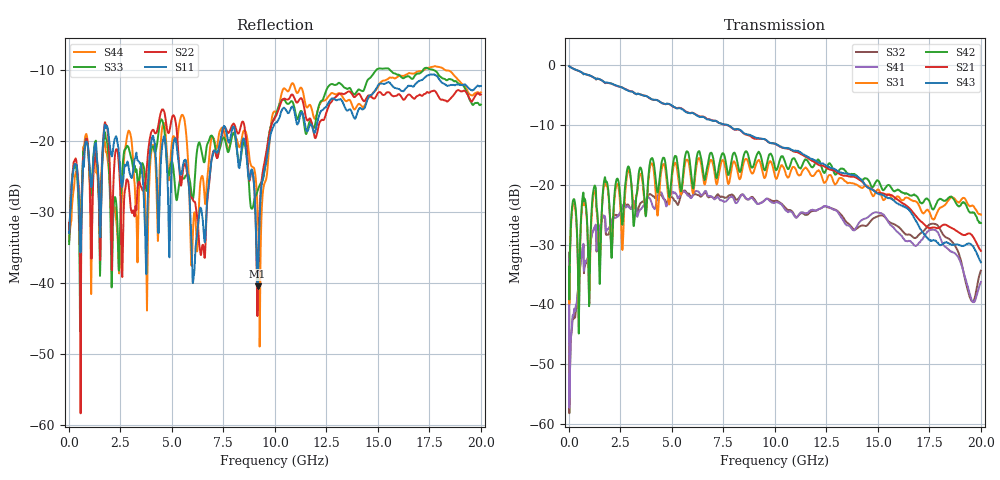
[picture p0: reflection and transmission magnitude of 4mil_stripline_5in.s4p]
! FILE: C:\Archive\Backplane\4-mil striplines\4mil_stripline_5in.s4p
! SMA ->1inch 21mil width microstrip -> 5 inch 4-mil width stripline -> 1 inch 21mil width microstrip -> SMA
! Port 1 -> Port 2, Port 3 -> Port 4
! 10/8/08
# MHz S DB R 50.00
! FREQ  S11  S12  S13  S14
!  S21  S22  S23  S24
!  S31  S32  S33  S34
!  S41  S42  S43  S44
!  DB  ANG  DB  ANG  DB  ANG  DB  ANG
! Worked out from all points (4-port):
!   2000 points, 10 MHz to 20 GHz, reference 50 ohm
!   strongest paths, dB at 10 MHz, 5.01 GHz, 10.01 GHz, 15.01 GHz, 20 GHz:
!     S43: -0.2, -6.8, -13.1, -21.5, -33.0
!     S21: -0.2, -6.8, -13.2, -21.4, -31.0
!     S42: -33.7, -17.7, -17.3, -19.3, -26.4
!     S31: -34.4, -18.5, -18.7, -20.8, -25.0
!     S41: -32.4, -21.3, -23.0, -24.6, -36.2
!     S32: -31.4, -22.1, -22.7, -25.2, -34.4
!   lowest |S11| = -40.5 dB at 9.16 GHz (marker M1), VSWR 1.02, Z = 49.1 - j0.0878 ohm
!   |S11| at or under -10 dB: start of sweep to end of sweep
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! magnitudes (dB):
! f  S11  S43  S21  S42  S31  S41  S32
! 10 MHz  -32.8  -0.2  -0.2  -33.7  -34.4  -32.4  -31.4
! 4.55 GHz  -20.1  -6.4  -6.4  -15.6  -16.7  -21.8  -22.1
! 6.51 GHz  -31.5  -8.7  -8.6  -17.8  -18.7  -21.6  -21.7
! 8.43 GHz  -19.9  -11.2  -11.3  -16.1  -17.2  -21.6  -21.6
! 9.16 GHz  -40.5  -12.2  -12.3  -14.7  -16.0  -23.2  -23.2
! 10.41 GHz  -15.3  -13.8  -13.8  -15.5  -17.0  -23.7  -23.5
! 20 GHz  -12.2  -33.0  -31.0  -26.4  -25.0  -36.2  -34.4
